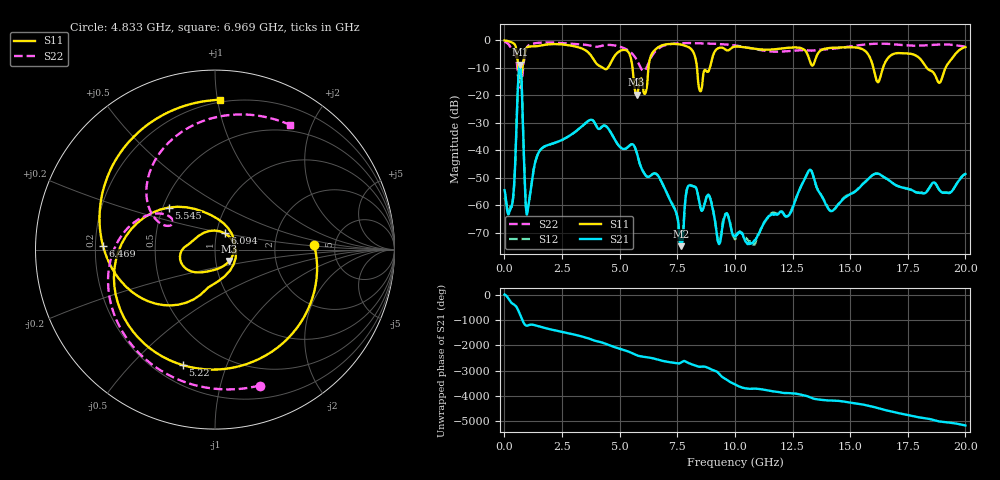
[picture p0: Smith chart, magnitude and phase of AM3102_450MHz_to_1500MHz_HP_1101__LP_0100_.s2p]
!Agilent Technologies,E8364B,MY43040894,A.07.50.67
!Agilent E8364B: A.07.50.67
!Date: Thursday, January 11, 2018 06:38:12
!Correction: S11(Full 2 Port(1,2))
!S21(Full 2 Port(1,2))
!S12(Full 2 Port(1,2))
!S22(Full 2 Port(1,2))
!S2P File: Measurements: S11, S21, S12, S22:
# Hz S  dB  R 50
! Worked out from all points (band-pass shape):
!   1601 points, 10 MHz to 20 GHz, reference 50 ohm
!   highest |S21| = -8.90 dB at 684.7 MHz (marker M1); lowest = -74.9 dB at 7.669 GHz (marker M2)
!   |S21| within 3 dB of the highest: 624.3 MHz to 726.2 MHz (101.9 MHz wide, 15.1 % of centre)
!   lowest |S11| = -19.8 dB at 5.732 GHz (marker M3), VSWR 1.23, Z = 58.2 - j7.38 ohm
!   |S11| at or under -10 dB: 5.558 GHz to 6.249 GHz (691.5 MHz wide, 11.7 % of centre); 8.357 GHz to 8.915 GHz (558.5 MHz wide, 6.47 % of centre); 18.32 GHz to 19.14 GHz (818.9 MHz wide, 4.37 % of centre)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
!   |S22| runs from -17.3 to -0.4 dB; largest |S21 - S12| = 0.0017
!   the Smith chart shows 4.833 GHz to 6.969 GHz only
!   S11 on the Smith chart (normalised r, x): 4.833 GHz: 3.44, +0.28; 5.22 GHz: 0.31, -0.71; 5.545 GHz: 0.54, +0.29; 6.094 GHz: 1.09, +0.20; 6.469 GHz: 0.23, +0.02; 6.969 GHz: 0.18, +1.01
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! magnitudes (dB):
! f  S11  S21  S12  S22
! 10 MHz  -0.1  -54.5  -57.3  -0.4
! 347.3 MHz  -0.9  -59.1  -59.4  -3.4
! 684.7 MHz  -13.6  -8.9  -8.9  -17.2
! 1.01 GHz  -2.5  -62.0  -61.3  -2.2
! 1.534 GHz  -2.0  -40.2  -40.2  -0.9
! 3.346 GHz  -2.9  -31.4  -31.4  -1.5
! 4.833 GHz  -5.2  -36.7  -36.7  -2.0
! 5.22 GHz  -3.5  -39.5  -39.6  -3.0
! 5.545 GHz  -9.1  -37.8  -37.8  -4.9
! 5.732 GHz  -19.8  -40.6  -40.6  -7.0
! 6.094 GHz  -19.5  -48.8  -48.8  -10.9
! 6.469 GHz  -4.1  -48.5  -48.5  -4.8
! 6.682 GHz  -2.5  -49.4  -49.5  -3.0
! 6.969 GHz  -1.6  -54.1  -54.1  -1.8
! 7.669 GHz  -1.6  -74.9  -73.1  -1.1
! 8.068 GHz  -2.9  -52.8  -52.7  -1.0
! 8.506 GHz  -18.6  -60.9  -60.8  -1.1
! 10.01 GHz  -2.3  -71.3  -72.4  -1.9
! 13.34 GHz  -9.1  -47.9  -47.9  -3.8
! 14.19 GHz  -2.8  -62.1  -62.2  -3.2
! 16.68 GHz  -6.1  -50.9  -50.9  -1.3
! 20 GHz  -2.5  -48.6  -48.6  -2.3
